FUNCTION FC 75 : VOID
TITLE =BLOCK OVERLOAD
AUTHOR : Esposito
FAMILY : EGAL_srl
NAME : OVERLOAD
VERSION : 0.1

BEGIN
NETWORK
TITLE =CONDITIONS FOR OVERLOAD PRESS
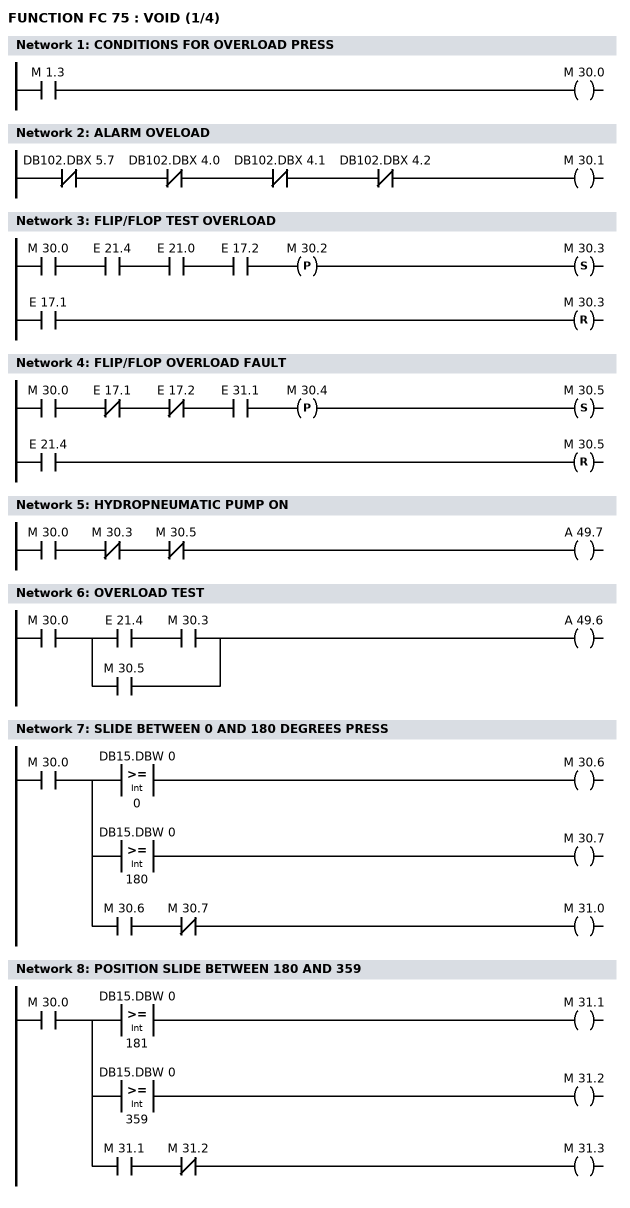
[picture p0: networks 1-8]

      U     M      1.3;
      =     M     30.0;
NETWORK
TITLE =ALARM OVELOAD

      UN    DB102.DBX    5.7;
      UN    DB102.DBX    4.0;
      UN    DB102.DBX    4.1;
      UN    DB102.DBX    4.2;
      =     M     30.1;
NETWORK
TITLE =FLIP/FLOP TEST OVERLOAD

      U     M     30.0;
      U     E     21.4;
      U     E     21.0;
      U     E     17.2;
      FP    M     30.2;
      S     M     30.3;
      U     E     17.1;
      R     M     30.3;
      NOP   0;
NETWORK
TITLE =FLIP/FLOP OVERLOAD FAULT

      U     M     30.0;
      UN    E     17.1;
      UN    E     17.2;
      U     E     31.1;
      FP    M     30.4;
      S     M     30.5;
      U     E     21.4;
      R     M     30.5;
      NOP   0;
NETWORK
TITLE =HYDROPNEUMATIC PUMP ON

      U     M     30.0;
      UN    M     30.3;
      UN    M     30.5;
      =     A     49.7;
NETWORK
TITLE =OVERLOAD TEST

      U     M     30.0;
      U(    ;
      U     E     21.4;
      U     M     30.3;
      O     M     30.5;
      )     ;
      =     A     49.6;
NETWORK
TITLE =SLIDE BETWEEN 0 AND 180 DEGREES PRESS

      U     M     30.0;
      =     L    218.0;
      U     L    218.0;
      U(    ;
      L     DB15.DBW    0;
      L     0;
      >=I   ;
      )     ;
      =     M     30.6;
      U     L    218.0;
      U(    ;
      L     DB15.DBW    0;
      L     180;
      >=I   ;
      )     ;
      =     M     30.7;
      U     L    218.0;
      U     M     30.6;
      UN    M     30.7;
      =     M     31.0;
NETWORK
TITLE =POSITION SLIDE BETWEEN 180 AND 359

      U     M     30.0;
      =     L    218.0;
      U     L    218.0;
      U(    ;
      L     DB15.DBW    0;
      L     181;
      >=I   ;
      )     ;
      =     M     31.1;
      U     L    218.0;
      U(    ;
      L     DB15.DBW    0;
      L     359;
      >=I   ;
      )     ;
      =     M     31.2;
      U     L    218.0;
      U     M     31.1;
      UN    M     31.2;
      =     M     31.3;
NETWORK
TITLE =CALL FC 105 - SCALING VALUES PIW292
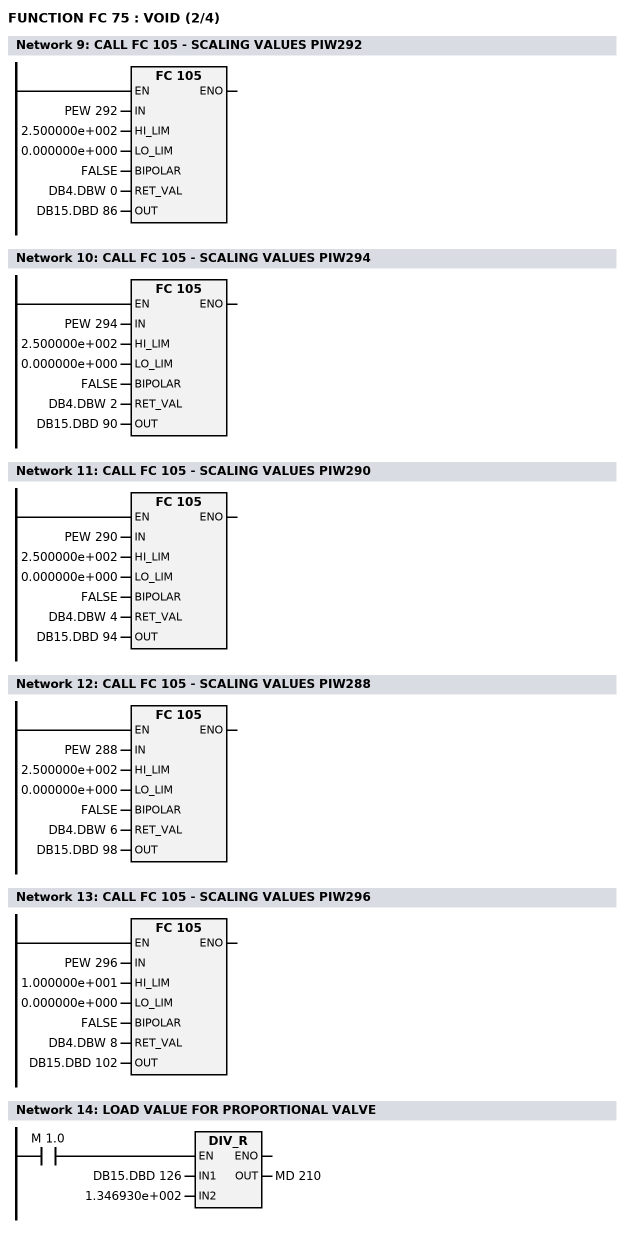
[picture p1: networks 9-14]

      CALL FC   105 (
           IN                       := PEW  292,
           HI_LIM                   := 2.500000e+002,
           LO_LIM                   := 0.000000e+000,
           BIPOLAR                  := FALSE,
           RET_VAL                  := DB4.DBW    0,
           OUT                      := DB15.DBD   86);

NETWORK
TITLE =CALL FC 105 - SCALING VALUES PIW294

      CALL FC   105 (
           IN                       := PEW  294,
           HI_LIM                   := 2.500000e+002,
           LO_LIM                   := 0.000000e+000,
           BIPOLAR                  := FALSE,
           RET_VAL                  := DB4.DBW    2,
           OUT                      := DB15.DBD   90);

NETWORK
TITLE =CALL FC 105 - SCALING VALUES PIW290

      CALL FC   105 (
           IN                       := PEW  290,
           HI_LIM                   := 2.500000e+002,
           LO_LIM                   := 0.000000e+000,
           BIPOLAR                  := FALSE,
           RET_VAL                  := DB4.DBW    4,
           OUT                      := DB15.DBD   94);

NETWORK
TITLE =CALL FC 105 - SCALING VALUES PIW288

      CALL FC   105 (
           IN                       := PEW  288,
           HI_LIM                   := 2.500000e+002,
           LO_LIM                   := 0.000000e+000,
           BIPOLAR                  := FALSE,
           RET_VAL                  := DB4.DBW    6,
           OUT                      := DB15.DBD   98);

NETWORK
TITLE =CALL FC 105 - SCALING VALUES PIW296

      CALL FC   105 (
           IN                       := PEW  296,
           HI_LIM                   := 1.000000e+001,
           LO_LIM                   := 0.000000e+000,
           BIPOLAR                  := FALSE,
           RET_VAL                  := DB4.DBW    8,
           OUT                      := DB15.DBD  102);

NETWORK
TITLE =LOAD VALUE FOR PROPORTIONAL VALVE

      U     M      1.0;
      SPBNB _001;
      L     DB15.DBD  126;
      L     1.346930e+002;
      /R    ;
      T     MD   210;
_001: NOP   0;
NETWORK
TITLE =CALL FC 106 - UNSCALING VALUES PQW 304
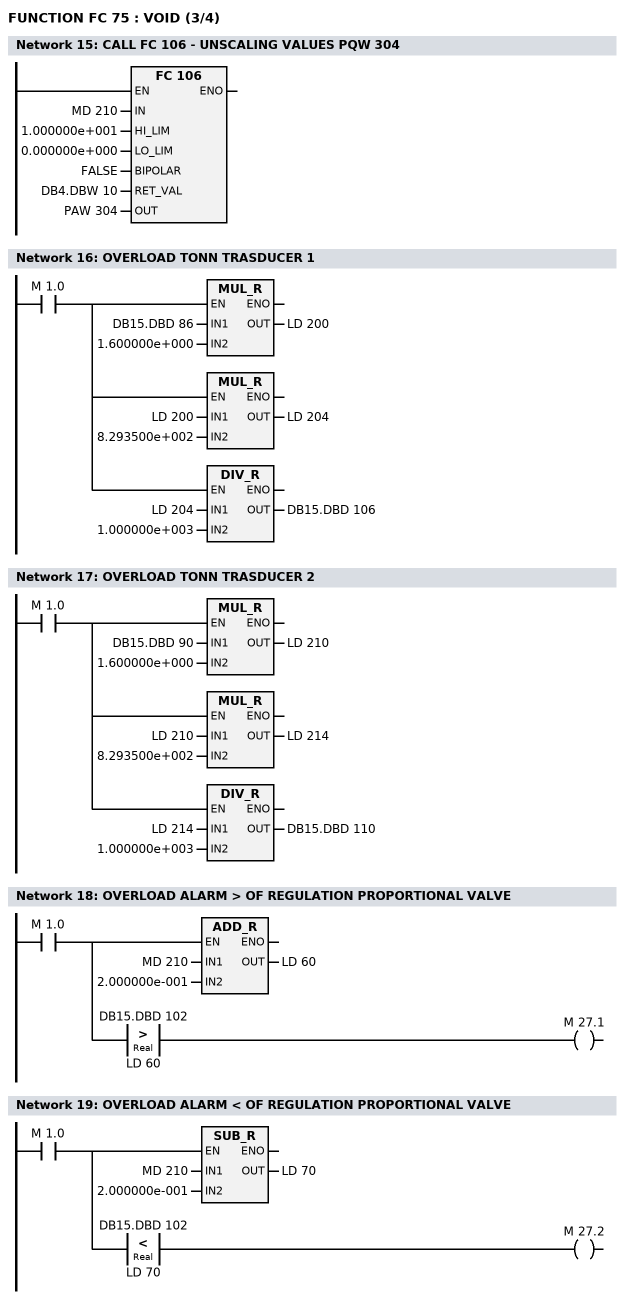
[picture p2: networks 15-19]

      CALL FC   106 (
           IN                       := MD   210,
           HI_LIM                   := 1.000000e+001,
           LO_LIM                   := 0.000000e+000,
           BIPOLAR                  := FALSE,
           RET_VAL                  := DB4.DBW   10,
           OUT                      := PAW  304);

NETWORK
TITLE =OVERLOAD TONN TRASDUCER 1

      U     M      1.0;
      =     L    218.0;
      U     L    218.0;
      SPBNB _002;
      L     DB15.DBD   86;
      L     1.600000e+000;
      *R    ;
      T     LD   200;
_002: NOP   0;
      U     L    218.0;
      SPBNB _003;
      L     LD   200;
      L     8.293500e+002;
      *R    ;
      T     LD   204;
_003: NOP   0;
      U     L    218.0;
      SPBNB _007;
      L     LD   204;
      L     1.000000e+003;
      /R    ;
      T     DB15.DBD  106;
_007: NOP   0;
NETWORK
TITLE =OVERLOAD TONN TRASDUCER 2

      U     M      1.0;
      =     L    218.0;
      U     L    218.0;
      SPBNB _00f;
      L     DB15.DBD   90;
      L     1.600000e+000;
      *R    ;
      T     LD   210;
_00f: NOP   0;
      U     L    218.0;
      SPBNB _013;
      L     LD   210;
      L     8.293500e+002;
      *R    ;
      T     LD   214;
_013: NOP   0;
      U     L    218.0;
      SPBNB _017;
      L     LD   214;
      L     1.000000e+003;
      /R    ;
      T     DB15.DBD  110;
_017: NOP   0;
NETWORK
TITLE =OVERLOAD ALARM > OF REGULATION PROPORTIONAL VALVE

      U     M      1.0;
      =     L    218.0;
      U     L    218.0;
      SPBNB _018;
      L     MD   210;
      L     2.000000e-001;
      +R    ;
      T     LD    60;
_018: NOP   0;
      U     L    218.0;
      U(    ;
      L     DB15.DBD  102;
      L     LD    60;
      >R    ;
      )     ;
      =     M     27.1;
NETWORK
TITLE =OVERLOAD ALARM < OF REGULATION PROPORTIONAL VALVE

      U     M      1.0;
      =     L    218.0;
      U     L    218.0;
      SPBNB _021;
      L     MD   210;
      L     2.000000e-001;
      -R    ;
      T     LD    70;
_021: NOP   0;
      U     L    218.0;
      U(    ;
      L     DB15.DBD  102;
      L     LD    70;
      <R    ;
      )     ;
      =     M     27.2;
NETWORK
TITLE =SET ALARM FOR PROPORTIONAL VALVE OVERLOAD
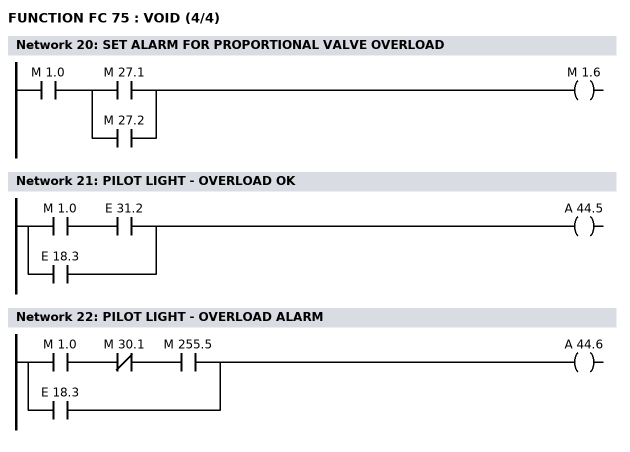
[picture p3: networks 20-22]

      U     M      1.0;
      U(    ;
      O     M     27.1;
      O     M     27.2;
      )     ;
      =     M      1.6;
NETWORK
TITLE =PILOT LIGHT - OVERLOAD OK

      U     M      1.0;
      U     E     31.2;
      O     E     18.3;
      =     A     44.5;
NETWORK
TITLE =PILOT LIGHT - OVERLOAD ALARM

      U     M      1.0;
      UN    M     30.1;
      U     M    255.5;
      O     E     18.3;
      =     A     44.6;
END_FUNCTION

